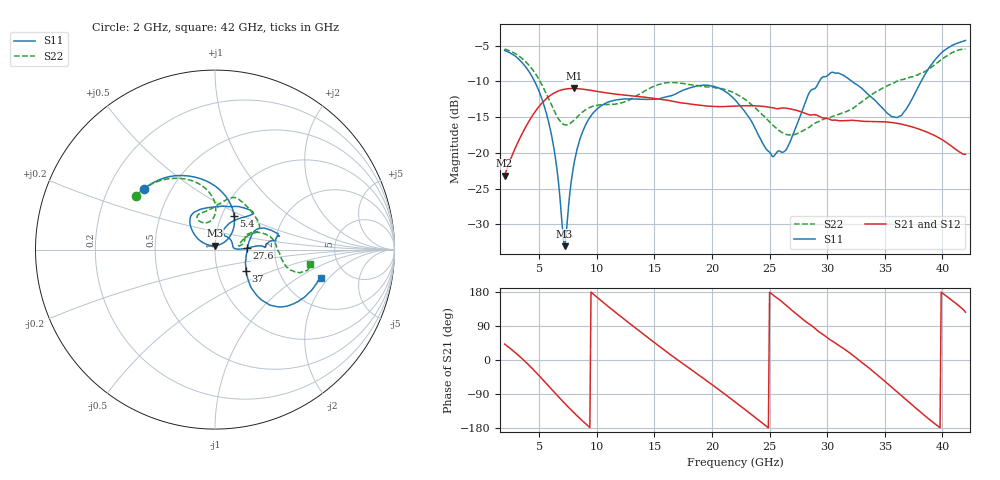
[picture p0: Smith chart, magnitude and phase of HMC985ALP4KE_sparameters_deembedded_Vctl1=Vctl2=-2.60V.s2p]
!s2p File: Measurements: S11, S21, S12, S22
# GHz S dB R 50.0
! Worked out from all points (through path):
!   401 points, 2 GHz to 42 GHz, reference 50 ohm
!   highest |S21| = -10.98 dB at 8 GHz (marker M1); lowest = -23.2 dB at 2 GHz (marker M2)
!   lowest |S11| = -33.1 dB at 7.2 GHz (marker M3), VSWR 1.05, Z = 49.8 + j2.2 ohm
!   |S11| at or under -10 dB: 4.607 GHz to 29.32 GHz (24.71 GHz wide, 146 % of centre); 32.17 GHz to 38.15 GHz (5.986 GHz wide, 17 % of centre)
!   |S22| runs from -17.5 to -5.4 dB; largest |S21 - S12| = 0.00027
!   S11 on the Smith chart (normalised r, x): 2 GHz: 0.35, +0.33; 5.4 GHz: 1.14, +0.45; 27.6 GHz: 1.43, +0.02; 37 GHz: 1.37, -0.35; 42 GHz: 3.28, -1.64
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2  -5.65 139.6  -23.19 42.0  -23.19 42.0  -5.46 145.6
3.6  -7.51 106.0  -17.07 1.3  -17.08 1.3  -6.90 118.5
5.4  -13.25 60.8  -12.76 -54.6  -12.76 -54.6  -10.99 91.8
6.3  -19.57 40.8  -11.62 -84.7  -11.62 -84.7  -14.10 89.9
7.2  -33.08 94.7  -11.09 -114.0  -11.09 -114.0  -16.07 103.4
8  -21.74 149.9  -10.98 -138.7  -10.98 -138.7  -15.45 115.9
8.7  -17.34 144.7  -11.06 -158.9  -11.06 -158.9  -14.38 119.6
10.1  -13.75 132.9  -11.40 163.6  -11.41 163.6  -13.31 115.6
12.2  -12.48 119.6  -11.88 111.9  -11.89 111.9  -12.98 98.1
15.4  -12.44 86.6  -12.47 36.8  -12.47 36.8  -10.41 72.8
18.2  -10.85 52.8  -13.18 -25.4  -13.19 -25.4  -10.46 54.7
22  -12.56 49.4  -13.44 -110.5  -13.45 -110.5  -11.68 23.5
25.3  -20.55 54.5  -13.68 171.6  -13.68 171.6  -16.16 17.7
26.4  -19.66 5.4  -13.74 145.2  -13.74 145.2  -17.40 11.8
27.6  -15.10 2.5  -14.17 114.5  -14.18 114.5  -17.13 8.8
28.7  -11.11 2.4  -14.68 89.5  -14.69 89.5  -16.10 11.2
31.1  -8.90 14.6  -15.51 36.8  -15.51 36.8  -14.54 23.9
33.3  -11.40 25.7  -15.59 -13.0  -15.60 -13.0  -12.52 23.7
35.4  -14.66 6.4  -15.71 -66.5  -15.71 -66.5  -10.48 16.1
37  -13.53 -34.9  -16.20 -108.6  -16.20 -108.6  -9.50 7.3
39.7  -6.34 -41.5  -17.89 -176.4  -17.90 -176.4  -7.22 -15.2
42  -4.25 -14.8  -20.20 126.1  -20.21 126.1  -5.42 -8.6
